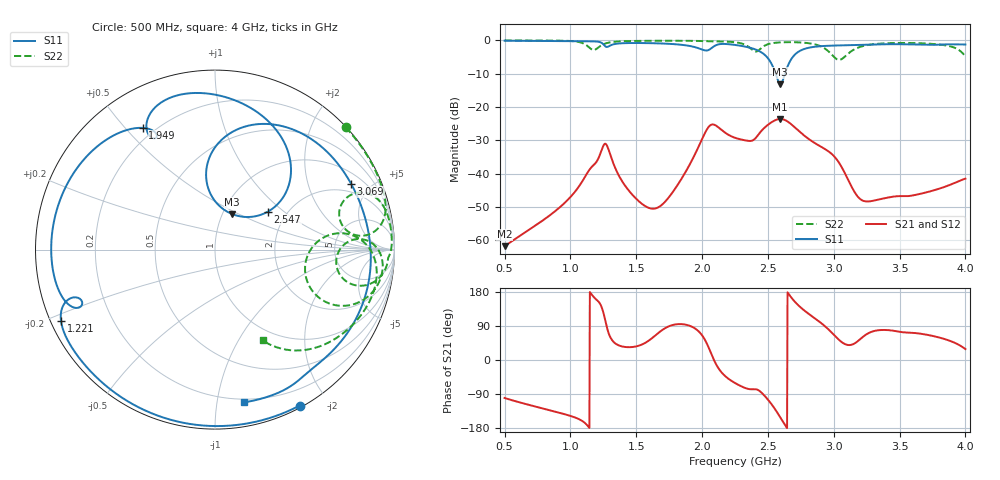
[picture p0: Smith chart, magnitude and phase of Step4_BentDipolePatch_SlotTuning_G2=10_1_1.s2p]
! TOUCHSTONE file generated by CST MICROWAVE STUDIO
! Date and time: Wed May 20 23:31:12 2020
! Project name: DualBand_DualMode_Antenna_FD_SteppedDesign.cst
! Parameters = {FPL=20; FPW=20; L=50; ST=10; SW=30; W=52; WF=7; ext=10; gap=1; inset=13}
! Header version: 2015
! Port assignment regex: !\s*Touchstone port\s*([0-9]+)\s*=\s*CST MWS port\s*([0-9]+)\s*\(\"(.*)\"\)(\s*mode\s*([0-9]+))?.*
! Touchstone port assignment:
! Touchstone port 1 = CST MWS port 1 ("")
! Touchstone port 2 = CST MWS port 2 ("")
# GHz S MA R 50
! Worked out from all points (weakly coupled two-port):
!   1006 points, 500 MHz to 4 GHz, reference 50 ohm
!   highest |S21| = -23.58 dB at 2.593 GHz (marker M1); lowest = -61.7 dB at 500 MHz (marker M2)
!   lowest |S11| = -13.2 dB at 2.593 GHz (marker M3), VSWR 1.56, Z = 55.6 + j23.1 ohm
!   |S11| at or under -10 dB: 2.559 GHz to 2.63 GHz (70.92 MHz wide, 2.73 % of centre)
!   |S22| runs from -5.9 to 0.0 dB; largest |S21 - S12| = 0.00019
!   S11 on the Smith chart (normalised r, x): 500 MHz: 0.02, -1.68; 1.221 GHz: 0.03, -0.22; 1.949 GHz: 0.16, +0.56; 2.547 GHz: 1.60, +0.78; 3.069 GHz: 1.51, +3.80; 4 GHz: 0.17, -1.20
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0.5  0.9886 -61.6  0.0008211 -100.2  0.0008211 -100.2  0.9968 43.1
0.7905  0.9816 -97.4  0.001998 -128.0  0.001998 -128.0  0.9955 24.1
1.0845  0.9701 -134.4  0.007395 -159.8  0.007418 -160.0  0.9212 7.7
1.144  0.9676 -142.5  0.01147 -179.1  0.01139 -179.8  0.7778 6.2
1.221  0.9449 -155.3  0.01868 150.5  0.01867 150.8  0.8076 21.9
1.27  0.8009 -160.0  0.02783 96.2  0.02781 96.2  0.9032 20.3
1.4555  0.912 -176.3  0.005234 33.9  0.005222 33.7  0.9782 12.2
1.669  0.9014 156.6  0.003153 71.7  0.003148 71.7  0.9867 6.6
1.949  0.7881 120.7  0.02015 82.6  0.02015 82.6  0.982 0.2
2.0715  0.7647 119.8  0.05449 14.9  0.05449 14.9  0.9663 -2.6
2.25  0.8543 86.9  0.03462 -60.7  0.03462 -60.7  0.9372 -8.9
2.4005  0.7366 60.9  0.03331 -76.8  0.03331 -76.9  0.6812 -7.1
2.5475  0.3632 35.7  0.06242 -126.3  0.06242 -126.3  0.9164 -0.8
2.593  0.2199 64.0  0.06625 -150.8  0.06625 -150.8  0.9327 -3.4
2.67  0.495 94.4  0.05673 168.3  0.05673 168.3  0.9399 -7.4
2.8345  0.7911 59.2  0.03072 115.5  0.03072 115.5  0.8906 -17.1
2.957  0.8297 40.2  0.02188 81.7  0.02188 81.7  0.6928 -25.3
3.069  0.8423 25.8  0.0117 45.1  0.0117 45.1  0.5383 0.8
3.2125  0.8578 9.0  0.00403 58.4  0.004026 58.4  0.8119 4.0
3.419  0.8758 -15.0  0.004428 78.6  0.004426 78.6  0.9078 -7.2
3.797  0.8616 -55.8  0.00594 59.7  0.005942 59.7  0.8687 -29.8
4  0.8667 -79.1  0.008458 28.9  0.008458 28.9  0.571 -62.3
